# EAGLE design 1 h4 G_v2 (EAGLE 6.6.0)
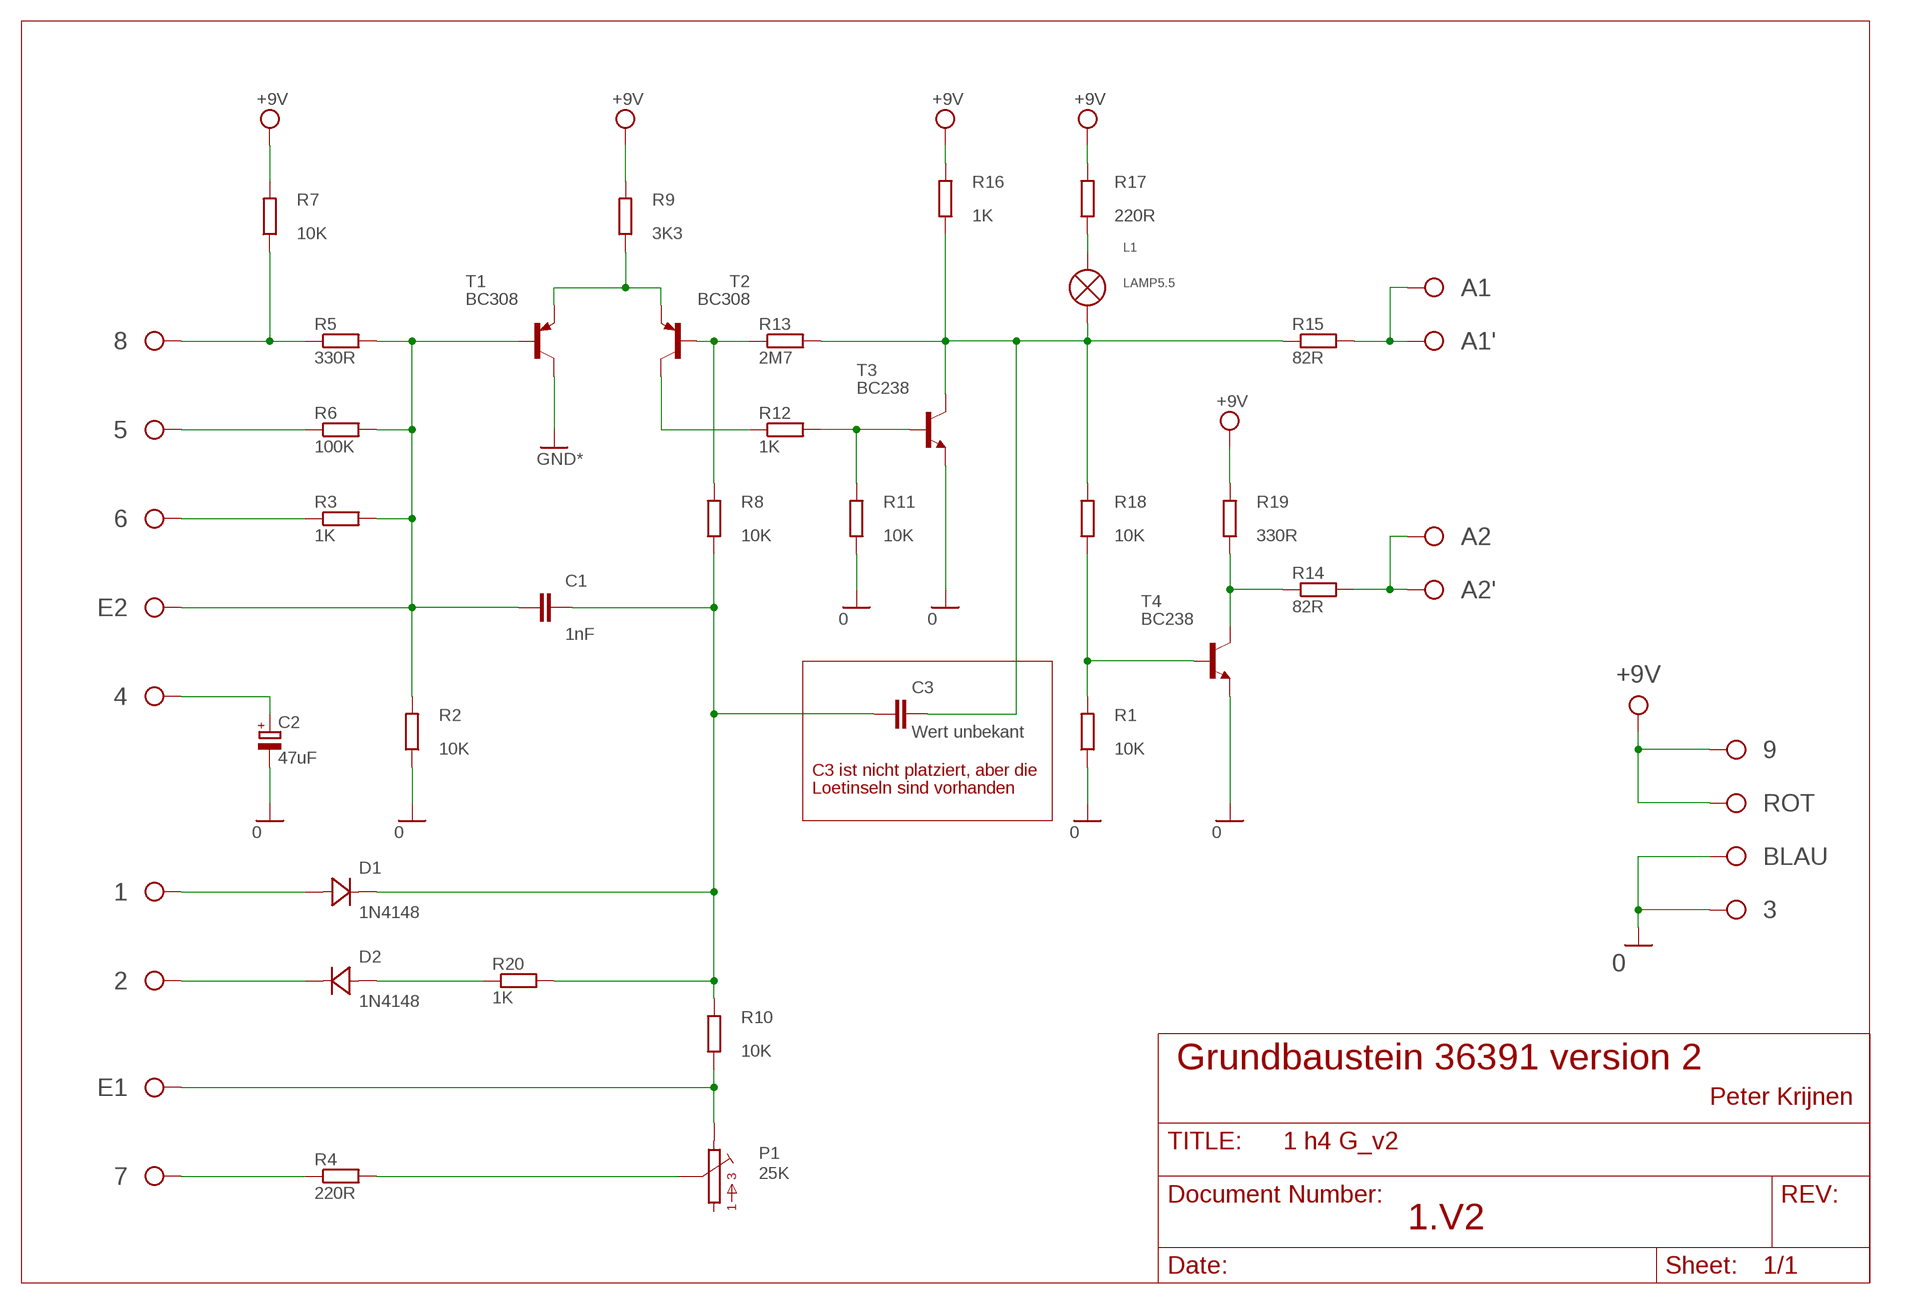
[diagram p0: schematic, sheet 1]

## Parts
1  PIN_2  [PIN_2]
2  PIN_2  [PIN_2]
3  PIN_2  [PIN_2]
4  PIN_2  [PIN_2]
5  PIN_2  [PIN_2]
6  PIN_2  [PIN_2]
7  PIN_2  [PIN_2]
8  PIN_2  [PIN_2]
9  PIN_2  [PIN_2]
A1  PIN_2  [PIN_2]
A1'  PIN_2  [PIN_2]
A2  PIN_2  [PIN_2]
A2'  PIN_2  [PIN_2]
BLAU  BLAU  [BLAU]
C1  1nF  C-EU025-025X050  [C025-025X050]
C2  47uF  CPOL-EUE2.5-7  [E2,5-7]
C3  Wert unbekant  C-EU025-025X050  [C025-025X050]
D1  1N4148  DIODE-7.5  [D-7.5]
D2  1N4148  DIODE-7.5  [D-7.5]
E1  PIN_2  [PIN_2]
E2  PIN_2  [PIN_2]
L1  LAMP5.5  [LAMP]
P1  25K  POT_FT41  [POT_FT4]
R1  10K  R-EU_0207/12  [0207/12]
R2  10K  R-EU_0207/12  [0207/12]
R3  1K  R-EU_0207/12  [0207/12]
R4  220R  R-EU_0207/15  [0207/15]
R5  330R  R-EU_0207/12  [0207/12]
R6  100K  R-EU_0207/12  [0207/12]
R7  10K  R-EU_0207/12  [0207/12]
R8  10K  R-EU_0207/12  [0207/12]
R9  3K3  R-EU_0207/12  [0207/12]
R10  10K  R-EU_0207/12  [0207/12]
R11  10K  R-EU_0207/12  [0207/12]
R12  1K  R-EU_0207/12  [0207/12]
R13  2M7  R-EU_0207/12  [0207/12]
R14  82R  R-EU_0207/15  [0207/15]
R15  82R  R-EU_0207/15  [0207/15]
R16  1K  R-EU_0207/12  [0207/12]
R17  220R  R-EU_0207/12  [0207/12]
R18  10K  R-EU_0207/12  [0207/12]
R19  330R  R-EU_0207/12  [0207/12]
R20  1K  R-EU_0207/12  [0207/12]
ROT  ROT  [ROT]
T1  BC308  BC557  [TO92]
T2  BC308  BC557  [TO92]
T3  BC238  [TO92]
T4  BC238  [TO92]

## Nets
GND: 3.P$1 BLAU.P$1 C2.- R1.1 R2.1 R11.1 T1.3(C) T3.1(E) T4.1(E) ; supply symbol labelled GND*, 0
N$1: 8.P$1 R5.1 R7.1
N$2: R12.1 T2.3(C)
N$3: 5.P$1 R6.1
N$4: 6.P$1 R3.1
N$5: C1.2 E2.P$1 R2.2 R3.2 R5.2 R6.2 T1.2(B)
N$6: 7.P$1 R4.1
N$7: E1.P$1 P1.P$3 R10.1
N$8: P1.P$2 R4.2
N$9: 1.P$1 D1.A
N$10: R9.1 T1.1(E) T2.1(E)
N$11: C1.1 C3.2 D1.K(C) R8.1 R10.2 R20.2
N$12: R8.2 R13.1 T2.2(B)
N$13: C3.1 L1.P$2 R13.2 R15.1 R16.1 R18.2 T3.3(C)
N$14: 4.P$1 C2.+
N$15: 2.P$1 D2.K(C)
N$16: R11.2 R12.2 T3.2(B)
N$17: R1.2 R18.1 T4.2(B)
N$18: D2.A R20.1
N$19: R14.1 R19.1 T4.3(C)
N$20: L1.P$1 R17.1
N$21: A1'.P$1 A1.P$1 R15.2
N$23: A2'.P$1 A2.P$1 R14.2
VCC: 9.P$1 R7.2 R9.2 R16.2 R17.2 R19.2 ROT.P$1 ; supply symbol labelled +9V

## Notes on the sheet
- C3 ist nicht platziert, aber die
- Loetinseln sind vorhanden
- Grundbaustein 36391 version 2
- Peter Krijnen
- 1.V2

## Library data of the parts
1-9 A1 A1' A2 A2' E1 E2 = ft_spec:PIN_2
BLAU = ft_spec:BLAU
C1 C3 = rcl:C-EU: CAPACITOR, European symbol
C2 = rcl:CPOL-EU: POLARIZED CAPACITOR, European symbol
D1 D2 = diode:DIODE-: DIODE
L1 = FT-SPEC:LAMP
P1 = FT-SPEC:POT_FT4
R1-R20 = rcl:R-EU_: RESISTOR, European symbol
ROT = ft_spec:ROT
T1 T2 = transistor-pnp:BC557: PNP TRANSISTOR
T3 T4 = transistor-npn:BC238: NPN TRANSISTOR

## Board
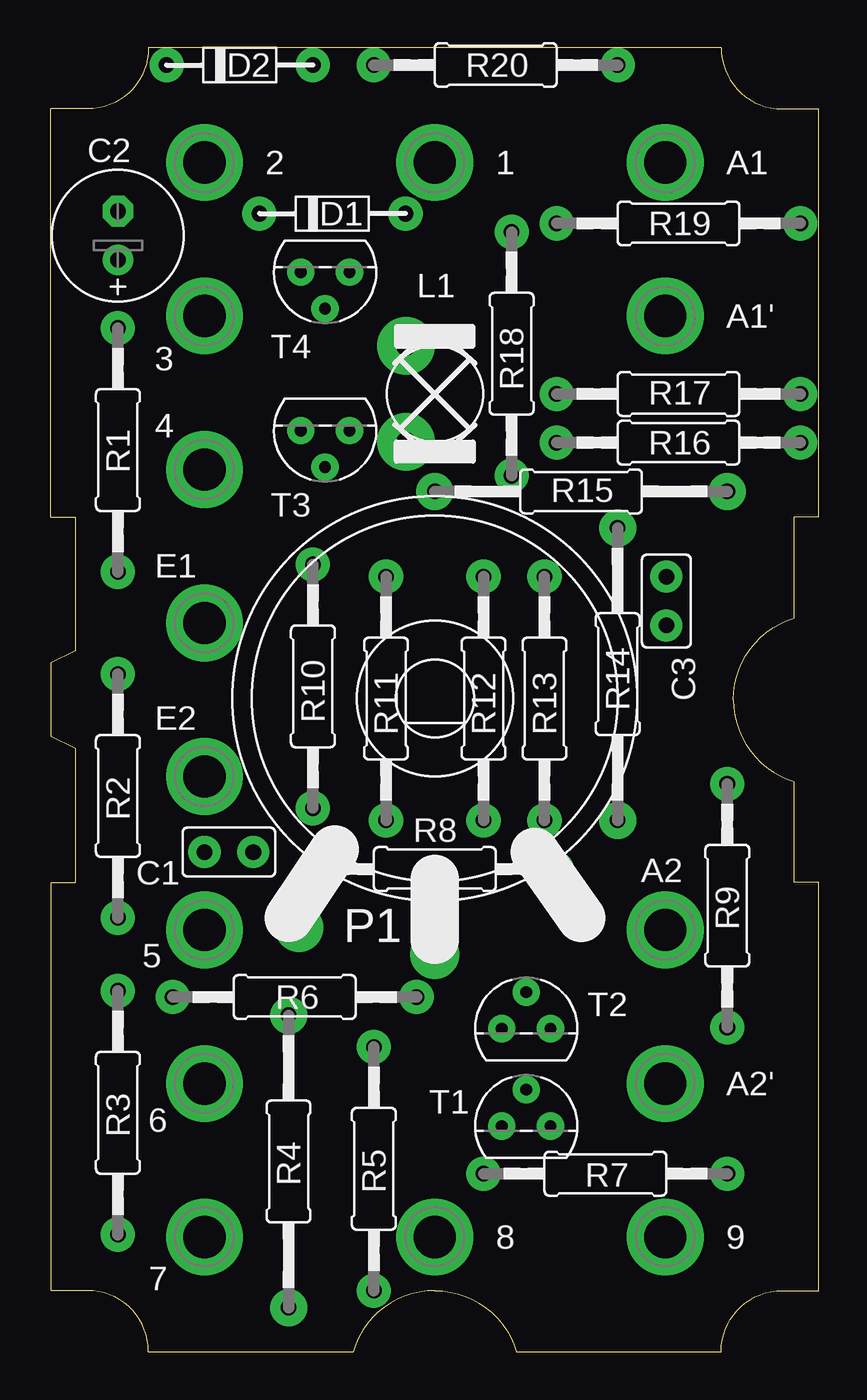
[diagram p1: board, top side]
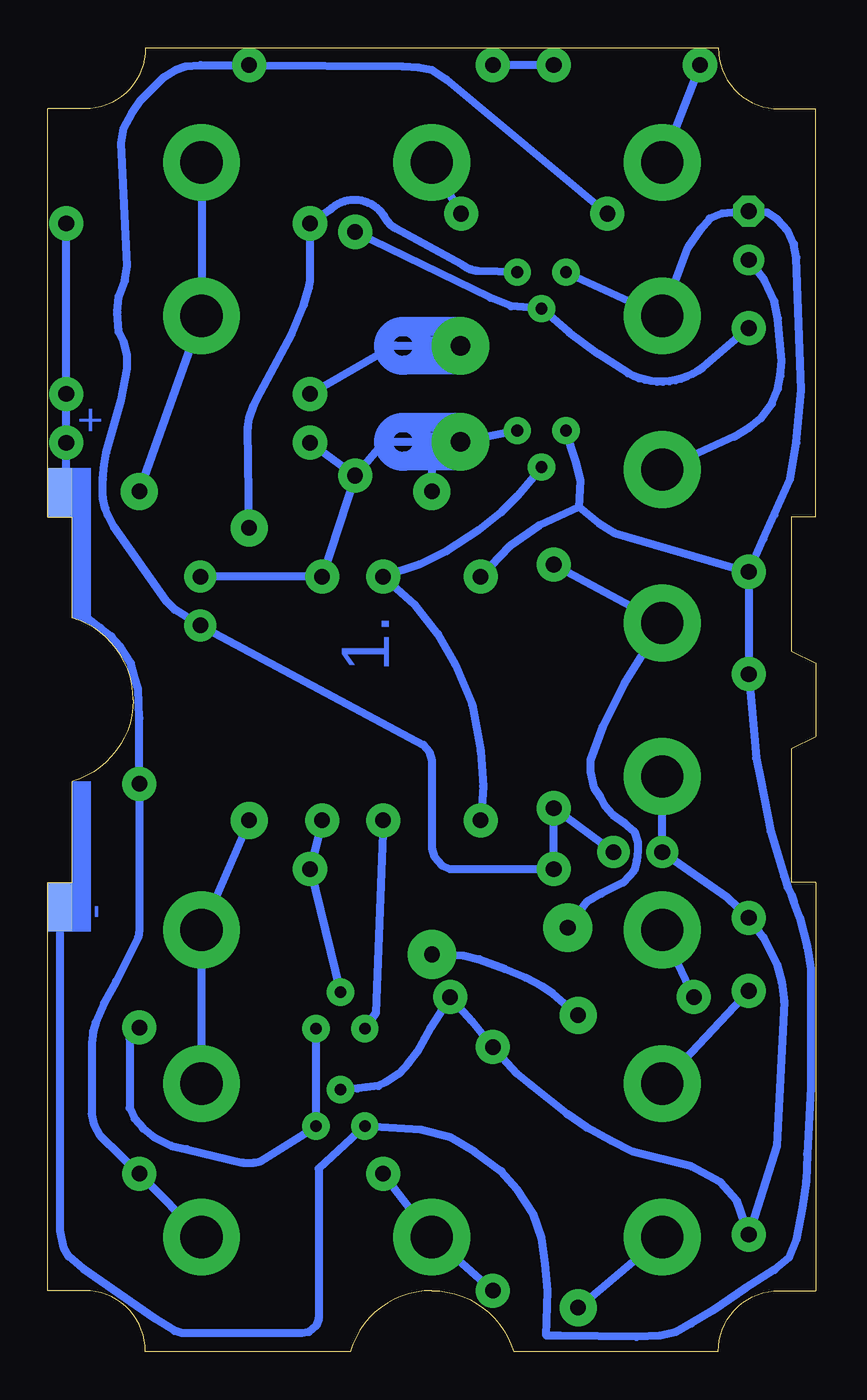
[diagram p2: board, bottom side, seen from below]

Size 40.01 x 67.94 mm. Coordinates in mm from the lower left corner, seen from the top.
Copper layers (1*16): Top 0.035mm / dielectric 1.5mm / Bottom 0.035mm
Design rules "default": minimum track width 10mil, minimum drill 24mil, track to track 8mil, track to pad 8mil, pad to pad 8mil, via to via 8mil, smd to smd 8mil, copper to edge 40mil, drill to drill 8mil, minimum pad ring 10mil, minimum via ring 8mil, stop-mask expansion 0mil, vias tented up to drill 0mil, thermal gap 10mil

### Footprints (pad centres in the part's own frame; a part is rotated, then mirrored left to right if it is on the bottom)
PIN_2 = drill 2.2 pad 4: P$1 0,0
BLAU = smd 2.54 x 1.27 bottom: P$1 0,0
C025-025X050 = drill 0.813 pad 1.676: 1 -1.27,0; 2 1.27,0
E2,5-7 = drill 0.813 pad 1.6: + -1.27,0 | drill 0.813 pad 1.6 octagon: - 1.27,0
D-7.5 = drill 0.813 pad 1.778: A -3.81,0; K 3.81,0
LAMP = drill 1.016 pad 3: P$1 -1.5,2.5; P$2 -1.5,-2.5
POT_FT4 = drill 0.813 pad 2.54: P$2 0,-13.335; P$3 -7.08,-11.938
0207/12 = drill 0.813 pad 1.778: 1 -6.35,0; 2 6.35,0
0207/15 = drill 0.813 pad 1.93: 1 -7.62,0; 2 7.62,0
ROT = smd 2.54 x 1.27 bottom: P$1 0,0
TO92 = drill 0.61 pad 1.422: 1 1.27,0; 2 0,1.905; 3 -1.27,0

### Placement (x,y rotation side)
1  20,61.98 0 top
2  8,61.98 0 top
3  8,53.98 0 top
4  8,45.97 0 top
5  8,21.97 0 top
6  8,13.97 0 top
7  8,5.97 0 top
8  20,5.97 0 top
9  32,5.97 0 top
A1  32,61.98 0 top
A1'  32,53.98 0 top
A2  32,21.97 0 top
A2'  32,13.97 0 top
BLAU  39.37,23.18 90 top
C1  9.27,26.04 180 top
C2  3.49,58.17 90 top
C3  32.07,39.12 270 top
D1  14.67,59.31 180 top
D2  9.84,67.06 180 top
E1  8,37.97 0 top
E2  8,29.97 0 top
L1  20,49.91 0 top
P1  20,34.04 0 top
R1  3.49,46.99 90 top
R2  3.49,28.96 270 top
R3  3.49,12.45 270 top
R4  12.38,9.91 90 top
R5  16.83,9.53 90 top
R6  12.7,18.48 0 top
R7  28.89,9.27 0 top
R8  20,25.15 0 top
R9  35.24,23.24 90 top
R10  13.65,34.67 270 top
R11  17.46,34.04 270 top
R12  22.54,34.04 90 top
R13  25.72,34.04 90 top
R14  29.53,35.31 270 top
R15  27.62,44.83 0 top
R16  32.7,47.37 0 top
R17  32.7,49.91 0 top
R18  24,52.01 270 top
R19  32.7,58.8 0 top
R20  23.18,67.06 0 top
ROT  39.37,44.77 90 top
T1  24.77,11.75 0 top
T2  24.77,16.83 0 top
T3  14.29,48.01 180 top
T4  14.29,56.26 180 top
U$2  [DIM_4070]  40.01,0 90 top

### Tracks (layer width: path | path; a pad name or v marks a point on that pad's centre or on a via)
GND
  Bottom 0.406: 12.32,44.01 12.26,45.4 12.51,46.42 T3.1 | 12.32,44.01 11.3,43.18 10.48,42.67 R1.1 | R1.1 2.73,42.35 2.16,43.62 1.33,45.47 1.02,47.37 0.76,50.1 1.02,57.02 1.14,57.72 1.46,58.42 1.97,58.99 2.54,59.37 C2.- 4.89,59.31 5.52,59.05 6.03,58.48 6.67,57.53 3.P$1 T4.1 | R1.1 R2.1 3.11,30.92 2.86,29.78 2.35,27.11 1.65,24.77 1.46,24.19 1.27,23.81 1.14,23.43 0.83,22.61 0.45,21.08 0.25,19.94 0.25,13.78 0.45,10.29 0.51,8.89 0.7,7.49 1.02,5.84 1.4,4.89 2.16,4.25 3.68,3.3 5.33,2.16 6.48,1.46 7.3,1.02 8.13,0.83 9.34,0.76 13.34,0.83 14.03,0.83 13.97,3.17 14.1,4.57 14.29,5.91 14.73,7.18 15.56,8.45 16.38,9.4 17.78,10.41 19.05,11.18 20.57,11.56 T1.3 25.91,9.53 25.91,1.71 26.04,1.33 26.42,1.02 26.8,0.95 33.02,0.95 33.4,1.08 34.42,1.71 38.16,4.32 38.92,4.95 39.18,5.4 39.37,6.29 BLAU.P$1 | R11.1 15.94,41.97 14.41,43.05 12.32,44.01
N$1
  Bottom 0.406: R5.1 8.P$1 R7.1
N$2
  Bottom 0.406: R12.1 22.92,17.65 T2.3
N$3
  Bottom 0.406: R6.1 5.P$1
N$4
  Bottom 0.406: R3.1 6.P$1
N$5
  Bottom 0.406: T1.2 23.88,13.72 23.43,13.78 22.8,13.84 22.42,14.03 21.72,14.48 21.21,15.05 20.77,15.62 20.38,16.32 20.07,16.89 R6.2 17.91,17.21 R5.2 15.56,14.48 14.86,13.91 12.95,12.38 11.94,11.68 10.67,10.99 9.53,10.41 6.48,9.65 4.95,8.83 4.13,7.87 R3.2 2.03,10.73 1.65,18.22 1.78,19.24 2.03,20.19 2.73,21.59 R2.2 4.64,23.69 C1.2 E2.P$1
N$6
  Bottom 0.406: R4.1 7.P$1
N$7
  Bottom 0.406: P1.P$3 12.89,22.1 11.94,23.43 11.62,23.62 11.18,23.88 10.03,24.45 9.46,25.08 9.34,25.59 9.27,26.1 9.27,26.54 9.46,27.11 9.97,27.56 10.6,28 10.99,28.45 11.24,28.89 11.56,29.4 11.75,30.23 11.75,30.8 11.11,32.58 9.97,34.8 E1.P$1 R10.1
N$8
  Bottom 0.406: R4.2 12.89,17.97 13.72,18.67 14.29,19.05 15.11,19.49 16.19,19.94 17.53,20.45 18.35,20.64 P1.P$2
N$9
  Bottom 0.406: D1.A 1.P$1
N$10
  Bottom 0.406: R9.1 35.75,16.32 35.75,12.7 35.5,12.13 35.05,11.62 34.48,11.18 33.59,10.73 32.77,10.54 29.84,9.84 29.27,9.84 28.96,9.91 T1.1 T2.1
N$11
  Bottom 0.406: D1.K 19.24,66.29 20,66.8 20.7,66.93 21.53,66.99 R20.2 32.07,67.06 32.83,66.99 33.34,66.8 33.97,66.42 35.18,65.22 35.62,64.58 36.07,63.75 36.2,62.99 35.88,56.58 36.01,55.82 36.32,54.99 36.39,54.17 36.32,53.15 36.07,52.64 35.88,51.94 35.88,51.24 36.2,49.59 36.96,46.86 37.08,46.23 37.15,45.47 37.15,44.51 37.02,43.94 36.89,43.62 36.58,42.99 33.85,39.12 33.4,38.67 C3.2 20.45,31.62 20.13,31.24 20,30.8 20,26.23 19.88,25.78 19.49,25.34 19.05,25.15 R8.1 R10.2 C1.1
N$12
  Bottom 0.406: R13.1 R8.2 T2.2
N$13
  Bottom 0.406: R18.2 R13.2 C3.1 | T3.3 L1.P$2 | L1.P$2 22.5,47.41 R18.2 | L1.P$2 20,47.41 R15.1 | R18.2 R16.1
N$14
  Bottom 0.406: C2.+ 2.67,55.82 2.16,54.74 1.97,53.85 1.78,51.63 1.84,50.86 1.97,50.16 2.29,49.4 2.86,48.64 3.43,48.2 4.25,47.69 4.P$1
N$15
  Bottom 0.406: D2.K 2.P$1
N$16
  Bottom 0.406: R11.2 17.34,29.46 17.46,31.3 17.91,33.72 18.8,35.81 19.68,37.4 20.89,38.92 R12.2 20.64,41.02 19.24,41.72 17.59,42.8 16.38,43.75 15.56,44.58 T3.2
N$17
  Bottom 0.406: R18.1 16.95,54.93 15.88,54.48 T4.2 arc-11 9.78,50.99 arc-72 5.65,51.5 R1.2
N$18
  Bottom 0.406: D2.A R20.1
N$19
  Bottom 0.406: R14.1 29.59,48.13 29.53,48.64 29.27,49.34 28.96,49.97 27.3,53.02 26.67,54.55 26.42,55.44 26.35,55.82 R19.1 25.34,59.5 arc105 22.42,59.05 arc-33 21.91,58.55 18.41,56.64 arc-38 17.59,56.33 T4.3
N$20
  Bottom 0.406: L1.P$1 21.87,52.41 21.91,52.45 R17.1
N$21
  Bottom 0.406: R15.2 A1'.P$1 A1.P$1
N$23
  Bottom 0.406: A2'.P$1 A2.P$1 R14.2
VCC
  Bottom 0.406: R19.2 R17.2 R16.2 39.05,44.83 ROT.P$1 38.54,44.01 38.48,38.99 38.48,38.35 37.78,38.1 37.27,37.72 36.7,37.27 36.26,36.77 35.69,35.88 35.5,35.12 35.31,34.54 35.24,33.02 R9.2 35.24,21.97 35.31,21.59 36.45,19.3 37.08,18.16 37.53,17.14 37.66,16.7 37.72,16.07 37.72,12.45 37.59,11.81 37.27,11.24 R7.2 9.P$1
(copper drawn outside any net)
  shapes: Bottom area x2

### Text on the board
Bottom: + | 1. | -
